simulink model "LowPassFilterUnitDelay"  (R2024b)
settings: Solver=FixedStepAuto  StartTime=0.0  StopTime=0.3  FixedStep=1e-3  RelTol=1e-3

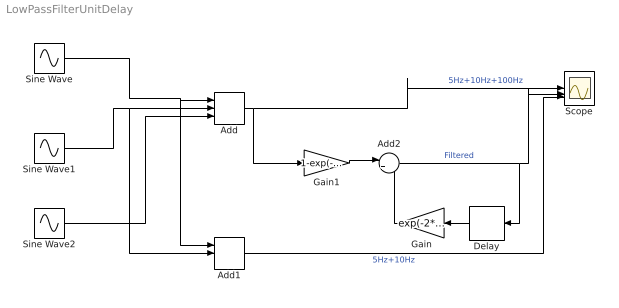
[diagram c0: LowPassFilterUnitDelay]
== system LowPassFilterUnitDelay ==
  Add : Sum  Inputs=+++
  Add1 : Sum  Inputs=+++
  Add2 : Sum  Inputs=|++
  Delay : Delay  DelayLength=1
  Gain : Gain  Gain=exp(-2*pi*20*1e-3)
  Gain1 : Gain  Gain=1-exp(-2*pi*20 * 1e-3)
  Scope : Scope  NumInputPorts=3
  Sine Wave : Sin  Frequency=2 * pi * 5  SampleTime=0
  Sine Wave1 : Sin  Frequency=2 * pi * 10  Phase=pi/4  SampleTime=0
  Sine Wave2 : Sin  Frequency=2 * pi * 100  Phase=pi/2  SampleTime=0
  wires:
  Sine Wave/1 -> Add1/1, Add/1
  Sine Wave1/1 -> Add1/2, Add/2
  Sine Wave2/1 -> Add/3
  Add/1 -> Gain1/1, Scope/1  "5Hz+10Hz+100Hz"
  Add1/1 -> Scope/3  "5Hz+10Hz"
  Gain1/1 -> Add2/1
  Add2/1 -> Delay/1, Scope/2  "Filtered"
  Delay/1 -> Gain/1
  Gain/1 -> Add2/2
